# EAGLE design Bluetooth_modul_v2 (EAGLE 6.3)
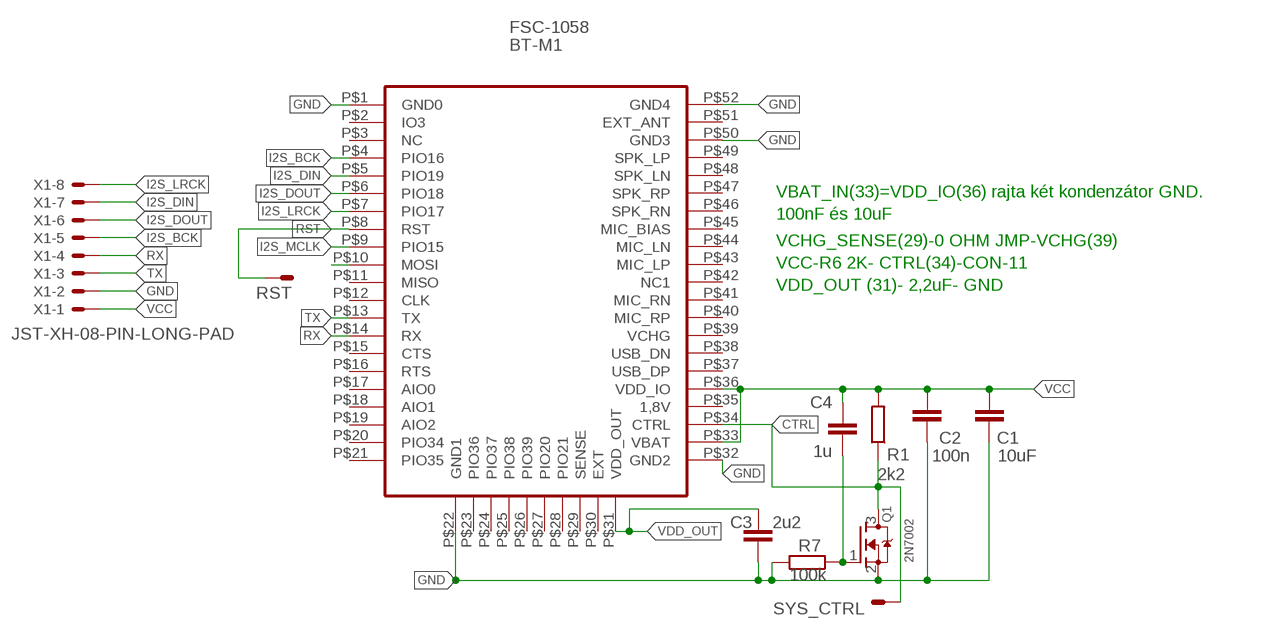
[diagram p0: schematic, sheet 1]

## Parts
BT-M1  FSC-1058  FSC-1054  [FSC-1054]
C1  10uF  C-EUC0805  [C0805]
C2  100n  C-EUC0603  [C0603]
C3  2u2  C-EUC0603  [C0603]
C4  1u  C-EUC0805  [C0805]
Q1  2N7002  MOSFET-NREFLOW  [SOT23]
R1  2k2  R-EU_R0603  [R0603]
R7  100k  R-EU_R0603  [R0603]
RST  PAD1  [PAD1]
SYS_CTRL  PAD1  [PAD1]
X1  JST-XH-08-PIN-LONG-PAD  [JST-XH-08-PACKAGE-LONG-PAD]

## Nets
CTRL: BT-M1.P$34(CTRL) Q1.3(D) R1.1 SYS_CTRL.1(S)
GND: BT-M1.P$1(GND0) BT-M1.P$22(GND1) BT-M1.P$32(GND2) BT-M1.P$50(GND3) BT-M1.P$52(GND4) C1.1 C2.1 C3.1 Q1.2(S) R7.2 X1.2
I2S_BCK: BT-M1.P$4(PIO16) X1.5
I2S_DIN: BT-M1.P$5(PIO19) X1.7
I2S_DOUT: BT-M1.P$6(PIO18) X1.6
I2S_LRCK: BT-M1.P$7(PIO17) X1.8
I2S_MCLK: BT-M1.P$9(PIO15)
N$5: C4.1 Q1.1(G) R7.1
N$7: BT-M1.P$10(MOSI)
RST: BT-M1.P$8(RST) RST.1(S)
RX: BT-M1.P$14(RX) X1.4
TX: BT-M1.P$13(TX) X1.3
VCC: BT-M1.P$33(VBAT) BT-M1.P$36(VDD_IO) C1.2 C2.2 C4.2 R1.2 X1.1
VDD_OUT: BT-M1.P$31(VDD_OUT) C3.2
Unconnected: BT-M1.P$2(IO3) BT-M1.P$3(NC) BT-M1.P$11(MISO) BT-M1.P$12(CLK) BT-M1.P$15(CTS) BT-M1.P$16(RTS) BT-M1.P$17(AIO0) BT-M1.P$18(AIO1) BT-M1.P$19(AIO2) BT-M1.P$20(PIO34) BT-M1.P$21(PIO35) BT-M1.P$23(PIO36) BT-M1.P$24(PIO37) BT-M1.P$25(PIO38) BT-M1.P$26(PIO39) BT-M1.P$27(PIO20) BT-M1.P$28(PIO21) BT-M1.P$29(SENSE) BT-M1.P$30(EXT) BT-M1.P$35(1,8V) BT-M1.P$37(USB_DP) BT-M1.P$38(USB_DN) BT-M1.P$39(VCHG) BT-M1.P$40(MIC_RP) BT-M1.P$41(MIC_RN) BT-M1.P$42(NC1) BT-M1.P$43(MIC_LP) BT-M1.P$44(MIC_LN) BT-M1.P$45(MIC_BIAS) BT-M1.P$46(SPK_RN) BT-M1.P$47(SPK_RP) BT-M1.P$48(SPK_LN) BT-M1.P$49(SPK_LP) BT-M1.P$51(EXT_ANT)

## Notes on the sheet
- VBAT_IN(33)=VDD_IO(36) rajta két kondenzátor GND.
- 100nF és 10uF
- VCHG_SENSE(29)-0 OHM JMP-VCHG(39)
- VCC-R6 2K- CTRL(34)-CON-11
- VDD_OUT (31)- 2,2uF- GND

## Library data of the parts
BT-M1 = SimonZs:FSC-1054
C1-C4 = resistor:C-EU: CAPACITOR, European symbol
Q1 = adafruit1:MOSFET-N: N-Channel Mosfet 2N7002E - 60V 260mA SOT23 [Digikey: 2N7002ET1GOSTR-ND] - REEL BSH103 - 30V 850mA SOT23 [Digikey: 568-5013-1-ND]
R1 R7 = resistor:R-EU_: RESISTOR, European symbol
RST SYS_CTRL = tuskesor:PAD1
X1 = JST XH Connectors v1-0:JST-XH-08-PIN: JST XH Connector 2 Pin Wire to board connector. Pitch: 2,54 mm, (0.100") Number of pins: 8 Created by Rembrandt Electronics www.rembrandtelectronics.com

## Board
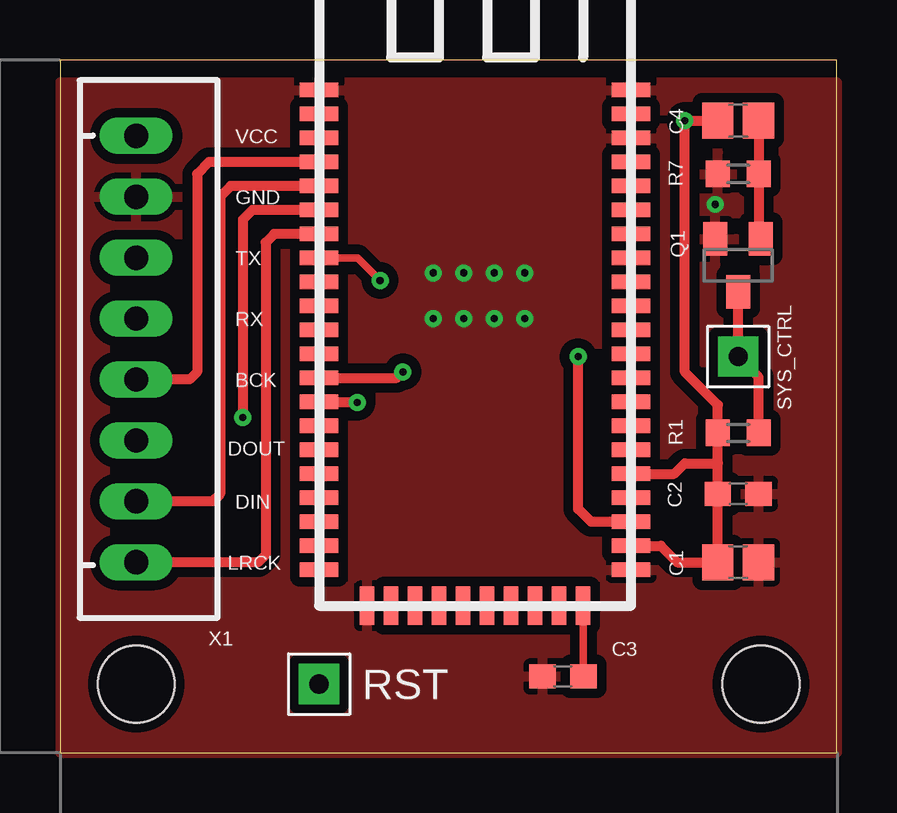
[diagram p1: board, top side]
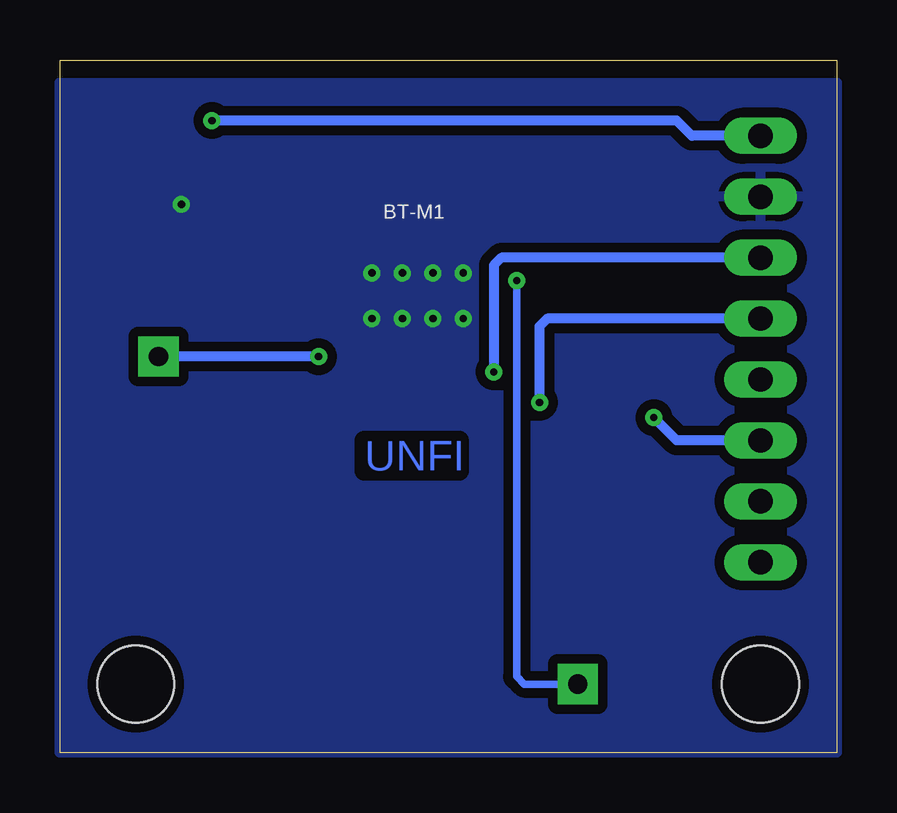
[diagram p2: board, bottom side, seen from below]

Size 32.37 x 28.88 mm. Coordinates in mm from the lower left corner, seen from the top.
Outline: 0,0 32.37,0 32.37,28.88 0,28.88 0,0
Copper layers (1*16): Top 0.035mm / dielectric 1.5mm / Bottom 0.035mm
Design rules "default *": minimum track width 10mil, minimum drill 0.6mm, track to track 8mil, track to pad 8mil, pad to pad 8mil, via to via 8mil, smd to smd 8mil, copper to edge 0mil, drill to drill 8mil, minimum pad ring 10mil, minimum via ring 8mil, stop-mask expansion 4mil, vias tented up to drill 0mil, thermal gap 10mil
Holes 3.2 mm at 3.17,2.86 29.21,2.86

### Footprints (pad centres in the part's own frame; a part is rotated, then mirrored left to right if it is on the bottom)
FSC-1054 = smd 1.6 x 0.6: P$1 0,0; P$2 0,-1; P$3 0,-2; P$4 0,-3; P$5 0,-4; P$6 0,-5; P$7 0,-6; P$8 0,-7; P$9 0,-8; P$10 0,-9; P$11 0,-10; P$12 0,-11; P$13 0,-12; P$14 0,-13; P$15 0,-14; P$16 0,-15; P$17 0,-16; P$18 0,-17; P$19 0,-18; P$20 0,-19; P$21 0,-20; P$32 13,-20; P$33 13,-19; P$34 13,-18; P$35 13,-17; P$36 13,-16; P$37 13,-15; P$38 13,-14; P$39 13,-13; P$40 13,-12; P$41 13,-11; P$42 13,-10; P$43 13,-9; P$44 13,-8; P$45 13,-7; P$46 13,-6; P$47 13,-5; P$48 13,-4; P$49 13,-3; P$50 13,-2; P$51 13,-1; P$52 13,0 | smd 0.6 x 1.6: P$22 2,-21.5; P$23 3,-21.5; P$24 4,-21.5; P$25 5,-21.5; P$26 6,-21.5; P$27 7,-21.5; P$28 8,-21.5; P$29 9,-21.5; P$30 10,-21.5; P$31 11,-21.5
C0805 = smd 1.3 x 1.5: 1 -0.85,0; 2 0.85,0
C0603 = smd 1.1 x 1: 1 -0.85,0; 2 0.85,0
SOT23 = smd 1 x 1.4: 1 -0.95,-1.1; 2 0.95,-1.1; 3 0,1.1
R0603 = smd 1 x 1.1: 1 -0.85,0; 2 0.85,0
PAD1 = drill 0.8 pad 1.676 square: 1 0,0
JST-XH-08-PACKAGE-LONG-PAD = drill 1.016 long: 1 -8.89,0; 2 -6.35,0; 3 -3.81,0; 4 -1.27,0; 5 1.27,0; 6 3.81,0; 7 6.35,0; 8 8.89,0

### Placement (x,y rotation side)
BT-M1  10.79,27.62 0 top
C1  28.26,7.94 180 top
C2  28.26,10.79 180 top
C3  20.95,3.17 0 top
C4  28.26,26.35 180 top
Q1  28.26,20.32 180 top
R1  28.26,13.34 180 top
R7  28.26,24.13 180 top
RST  10.79,2.86 90 top
SYS_CTRL  28.26,16.51 90 top
X1  3.17,16.83 270 top

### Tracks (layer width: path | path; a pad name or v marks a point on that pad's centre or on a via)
CTRL  (via drill 0.3)
  Top 0.406: BT-M1.P$34 22.13,9.62 21.59,10.16 v21.59,16.51 | R1.1 29.11,15.66 SYS_CTRL.1 Q1.3
  Bottom 0.406: v21.59,16.51 SYS_CTRL.1
GND  (via drill 0.3)
  other vias: 27.3,22.86 15.56,20 16.83,20 18.1,20 19.37,20 15.56,18.1 16.83,18.1 18.1,18.1 19.37,18.1
  pour Top (isolate 0.406): 0,0 32.39,0 32.39,27.94 0,27.94
  pour Bottom (isolate 0.406): 0,0 32.39,0 32.39,27.94 0,27.94
I2S_BCK
  Top 0.406: BT-M1.P$4 6.21,24.62 5.71,24.13 5.71,15.88 5.4,15.56 X1.5
I2S_DIN
  Top 0.406: BT-M1.P$5 7.11,23.62 6.67,23.18 6.67,10.79 6.35,10.48 X1.7
I2S_DOUT  (via drill 0.3)
  Top 0.406: BT-M1.P$6 8.02,22.62 7.62,22.22 v7.62,13.97
  Bottom 0.406: X1.6 6.67,13.02 v7.62,13.97
I2S_LRCK
  Top 0.406: BT-M1.P$7 8.92,21.62 8.57,21.27 8.57,8.25 8.26,7.94 X1.8
N$5
  Top 0.406: C4.1 R7.1 29.11,21.52 Q1.1
RST  (via drill 0.3)
  Top 0.305: BT-M1.P$8 12.4,20.62 v13.34,19.68
  Bottom 0.305: v13.34,19.68 13.34,3.17 13.02,2.86 RST.1
RX  (via drill 0.3)
  Top 0.406: BT-M1.P$14 12.37,14.62 v12.38,14.61
  Bottom 0.406: X1.4 12.06,18.1 12.38,17.78 v12.38,14.61
TX  (via drill 0.3)
  Top 0.406: BT-M1.P$13 14.04,15.62 v14.29,15.88
  Bottom 0.406: X1.3 13.97,20.64 14.29,20.32 v14.29,15.88
VCC  (via drill 0.3)
  Top 0.406: 27.41,12.06 C2.2 C1.2 25.72,7.94 25.03,8.62 BT-M1.P$33 | 27.41,12.06 R1.2 27.41,14.5 26.04,15.88 v26.04,26.35 C4.2 | BT-M1.P$36 25.59,11.62 26.04,12.06 27.41,12.06
  Bottom 0.406: X1.1 6.03,25.72 6.67,26.35 v26.04,26.35
VDD_OUT
  Top 0.305: BT-M1.P$31 21.79,3.18 C3.2

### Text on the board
Bottom: UNFI
tNames: VCC | GND | TX | RX | BCK | DOUT | DIN | LRCK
